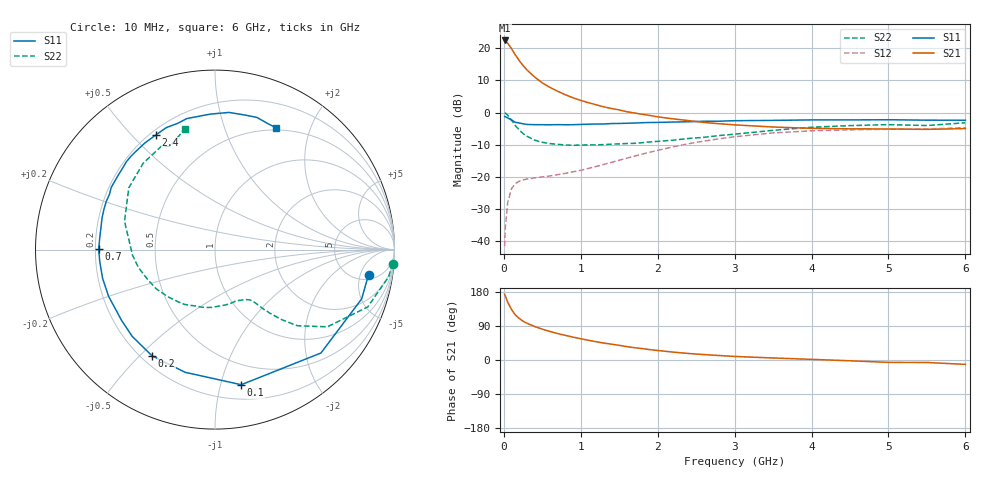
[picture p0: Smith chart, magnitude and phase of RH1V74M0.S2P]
! SIEMENS Small Signal Semiconductors
! BFR106
! Si NPN RF Bipolar Junction Transistor in SOT23
! VCE = 1.75 V  IC = 4 mA
! Common Emitter S-Parameters:  August  1996
# GHz  S  MA  R  50
!  f  S11  S21  S12  S22
! GHz  MAG  ANG  MAG  ANG  MAG  ANG  MAG  ANG
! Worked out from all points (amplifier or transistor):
!   36 points, 10 MHz to 6 GHz, reference 50 ohm
!   highest |S21| = 22.5 dB at 10 MHz (marker M1)
!   |S21| within 3 dB of that: start of sweep to 110.8 MHz
!   unconditionally stable (mu >= 1): 657.1 MHz to 2.287 GHz; 3.8 GHz to end of sweep
!   at 250 MHz: K = 0.45, MSG = 17.8 dB, |S12| = -21.0 dB
!   at 1.4 GHz: K = 1.19, MAG = 5.7 dB, |S12| = -15.5 dB
!   at 6 GHz: K = 1.02, MAG = -1.1 dB, |S12| = -4.7 dB
!   S11 on the Smith chart (normalised r, x): 10 MHz: 6.13, -6.92; 100 MHz: 0.32, -1.16; 200 MHz: 0.24, -0.54; 700 MHz: 0.21, +0.00; 2.4 GHz: 0.22, +0.59; 6 GHz: 0.47, +1.51
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0.01  0.8669 -9.3  13.27 173.7  0.0083 86.0  0.992 -4.5
0.02  0.862 -18.6  13.14 168.7  0.0167 80.9  0.9798 -8.8
0.05  0.8248 -44.3  12.04 152.6  0.0395 67.0  0.9089 -20.6
0.1  0.7669 -79.0  9.861 133.3  0.0654 52.0  0.7595 -34.5
0.15  0.7036 -103.7  7.871 118.8  0.0782 41.9  0.6257 -42.7
0.2  0.6878 -120.7  6.461 109.8  0.0853 37.0  0.5369 -46.5
0.25  0.6682 -133.7  5.381 102.3  0.0893 33.7  0.4699 -49.1
0.3  0.6533 -142.7  4.607 97.0  0.0923 32.4  0.4284 -50.8
0.4  0.6475 -156.3  3.577 88.4  0.0961 32.0  0.3721 -52.9
0.5  0.6464 -165.7  2.898 81.3  0.0995 33.2  0.3437 -54.9
0.6  0.6455 -173.9  2.463 75.2  0.103 35.4  0.3289 -57.8
0.7  0.6483 179.8  2.144 69.7  0.1077 38.1  0.3196 -61.4
0.9  0.6468 169.5  1.697 60.4  0.1195 44.1  0.3091 -68.7
1.1  0.6581 160.2  1.424 52.1  0.1348 49.2  0.3134 -78.0
1.3  0.6634 152.5  1.228 44.7  0.1558 53.0  0.3165 -87.5
1.6  0.6808 141.9  1.029 35.3  0.1951 56.0  0.3293 -103.1
2.2  0.7111 123.3  0.797 20.8  0.2923 53.0  0.3717 -135.1
2.4  0.7188 117.3  0.75 17.2  0.3269 50.2  0.3942 -146.5
3.5  0.7553 92.0  0.595 5.3  0.4815 29.6  0.5284 162.6
4.5  0.768 77.6  0.558 -2.1  0.5382 11.3  0.6262 129.6
5.5  0.7611 67.2  0.547 -6.5  0.5565 0.8  0.6277 113.6
6  0.7594 63.5  0.563 -11.6  0.5798 -6.6  0.6937 103.9
